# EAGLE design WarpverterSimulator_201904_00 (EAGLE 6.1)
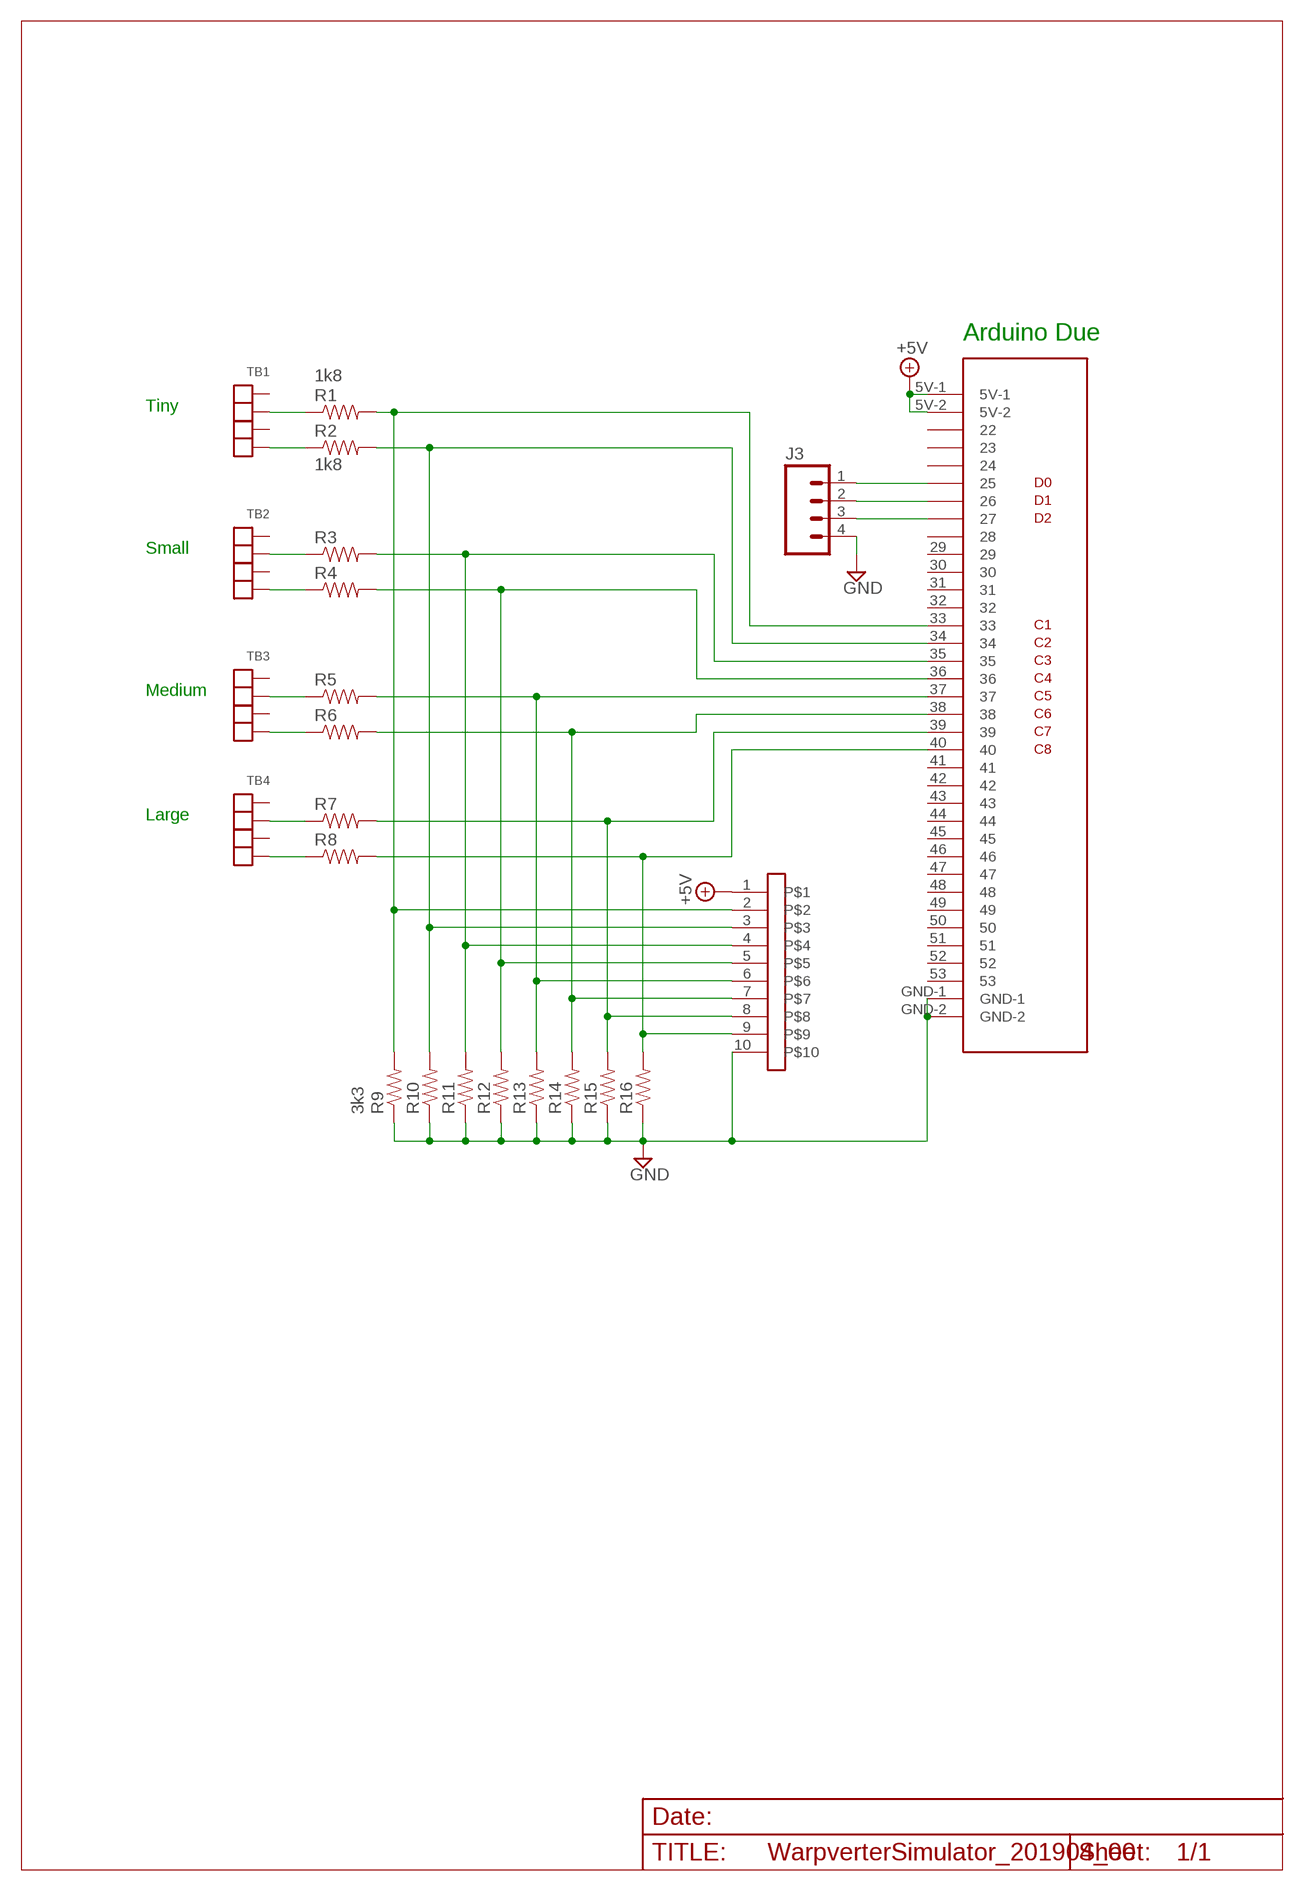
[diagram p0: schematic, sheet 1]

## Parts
J1  DUE-IDC38  [DUE-IDC38]
J2  SIL-STACK-10  [SIL-STACK-10]
J3  SIL4  [SIL4]
R1  1k8  R4  [AXIAL-0.4]
R2  1k8  R4  [AXIAL-0.4]
R3  R4  [AXIAL-0.4]
R4  R4  [AXIAL-0.4]
R5  R4  [AXIAL-0.4]
R6  R4  [AXIAL-0.4]
R7  R4  [AXIAL-0.4]
R8  R4  [AXIAL-0.4]
R9  3k3  R4  [AXIAL-0.4]
R10  R4  [AXIAL-0.4]
R11  R4  [AXIAL-0.4]
R12  R4  [AXIAL-0.4]
R13  R4  [AXIAL-0.4]
R14  R4  [AXIAL-0.4]
R15  R4  [AXIAL-0.4]
R16  R4  [AXIAL-0.4]
TB1  TB4381_SIL  [TB-381-SIL-4P]
TB2  TB4381_SIL  [TB-381-SIL-4P]
TB3  TB4381_SIL  [TB-381-SIL-4P]
TB4  TB4381_SIL  [TB-381-SIL-4P]

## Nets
+5V: J1.5V-1 J1.5V-2 J2.1
GND: J1.GND-1 J1.GND-2 J2.10 J3.4 R9.P$1 R10.P$1 R11.P$1 R12.P$1 R13.P$1 R14.P$1 R15.P$1 R16.P$1
N$1: R1.P$1 TB1.2 TB1.12
N$2: R2.P$1 TB1.4 TB1.14
N$3: R3.P$1 TB2.2 TB2.12
N$4: R4.P$1 TB2.4 TB2.14
N$5: R5.P$1 TB3.2 TB3.12
N$6: R6.P$1 TB3.4 TB3.14
N$7: R7.P$1 TB4.2 TB4.12
N$8: R8.P$1 TB4.4 TB4.14
N$9: J1.33 J2.2 R1.P$2 R9.P$2
N$10: J1.34 J2.3 R2.P$2 R10.P$2
N$11: J1.35 J2.4 R3.P$2 R11.P$2
N$12: J1.36 J2.5 R4.P$2 R12.P$2
N$13: J1.37 J2.6 R5.P$2 R13.P$2
N$14: J1.38 J2.7 R6.P$2 R14.P$2
N$15: J1.39 J2.8 R7.P$2 R15.P$2
N$16: J1.40 J2.9 R8.P$2 R16.P$2
N$18: J1.25 J3.1
N$19: J1.26 J3.2
N$20: J1.27 J3.3
Unconnected: J1.22 J1.23 J1.24 J1.28 J1.29 J1.30 J1.31 J1.32 J1.41 J1.42 J1.43 J1.44 J1.45 J1.46 J1.47 J1.48 J1.49 J1.50 J1.51 J1.52 J1.53 TB1.1 TB1.3 TB1.11 TB1.13 TB2.1 TB2.3 TB2.11 TB2.13 TB3.1 TB3.3 TB3.11 TB3.13 TB4.1 TB4.3 TB4.11 TB4.13

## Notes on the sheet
- Arduino Due
- Tiny
- Small
- Medium
- Large

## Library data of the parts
J1 = Andrew_Arduino:DUE-IDC38
J2 = Andrew_Connectors:SIL-STACK-10
J3 = Andrew_Connectors:SIL4
R1-R16 = Andrew Misc:R4
TB1-TB4 = Andrew_Connectors:TB4

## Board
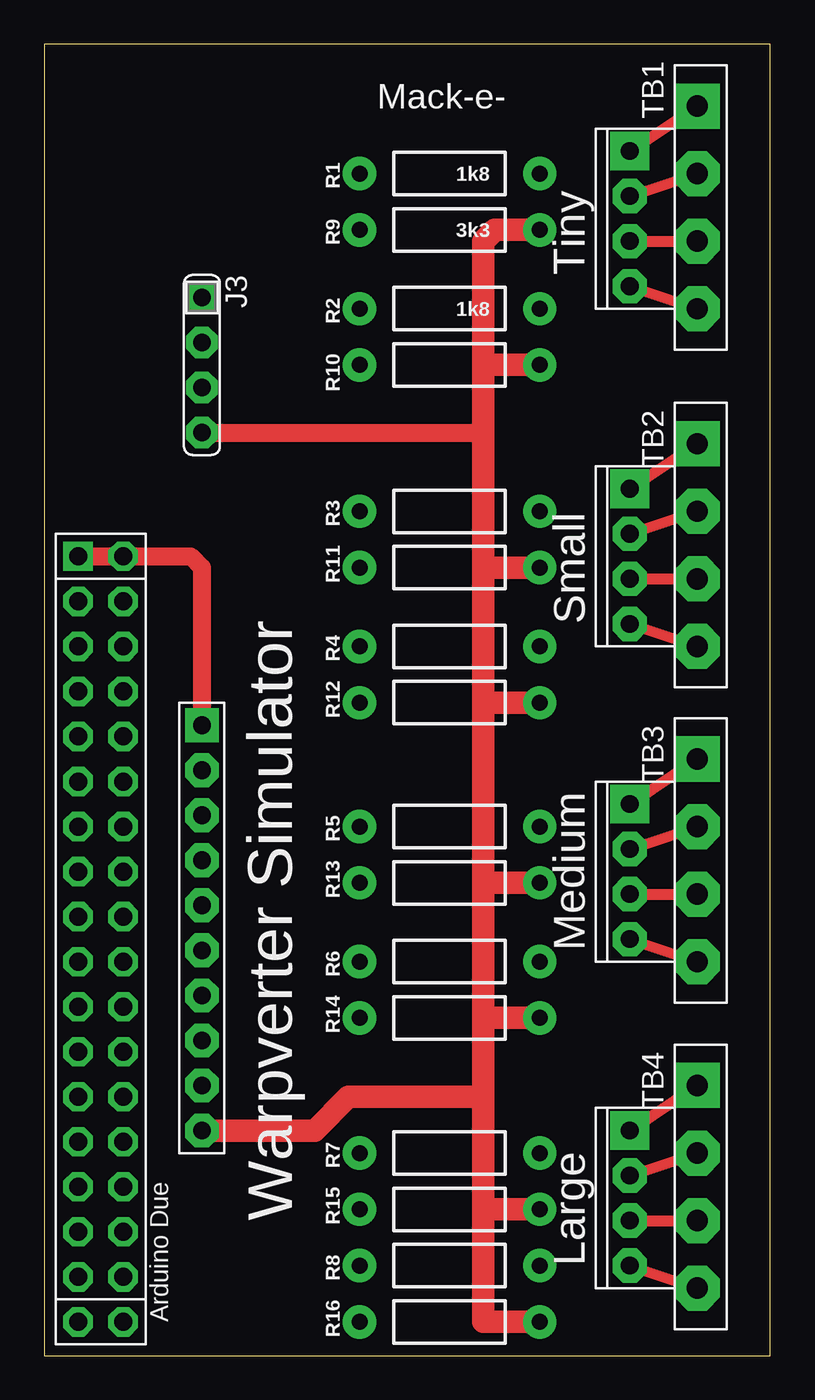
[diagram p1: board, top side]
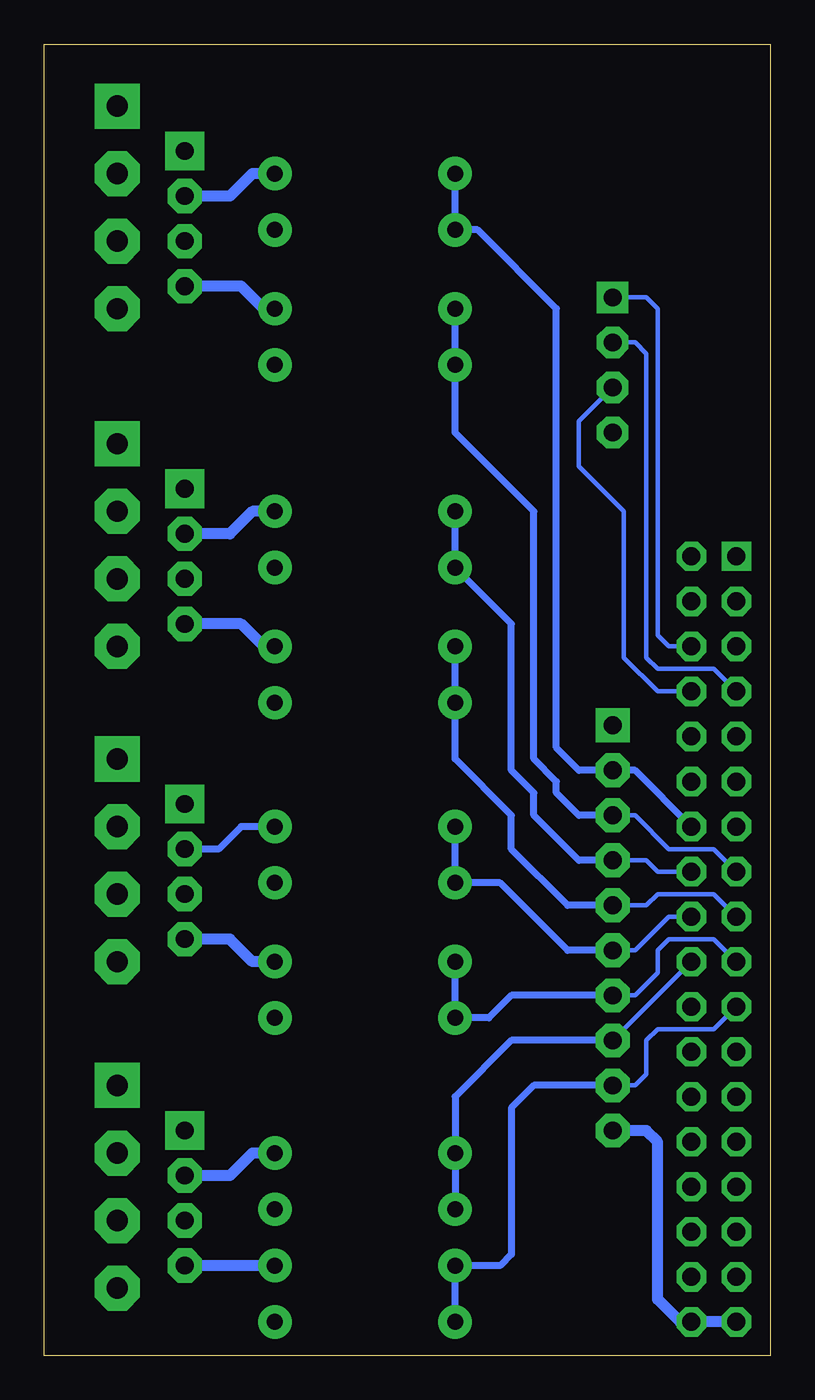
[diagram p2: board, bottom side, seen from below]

Size 40.95 x 73.97 mm. Coordinates in mm from the lower left corner, seen from the top.
Outline: 0,0 40.95,0 40.95,73.97 0,73.97 0,0
Copper layers (1*16): Top 0.035mm / dielectric 1.5mm / Bottom 0.035mm
Design rules: minimum track width 10mil, minimum drill 24mil, track to track 8mil, track to pad 8mil, pad to pad 8mil, via to via 8mil, smd to smd 8mil, copper to edge 40mil, drill to drill 8mil, minimum pad ring 10mil, minimum via ring 8mil, stop-mask expansion 4mil, vias tented up to drill 0mil, thermal gap 10mil

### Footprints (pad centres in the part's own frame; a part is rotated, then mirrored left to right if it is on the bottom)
DUE-IDC38 = drill 1.016 pad 1.651 square: 5V-1 0,2.54 | drill 1.016 pad 1.651 octagon: 5V-2 2.54,2.54; 22 0,0; 23 2.54,0; 24 0,-2.54; 25 2.54,-2.54; 26 0,-5.08; 27 2.54,-5.08; 28 0,-7.62; 29 2.54,-7.62; 30 0,-10.16; 31 2.54,-10.16; 32 0,-12.7; 33 2.54,-12.7; 34 0,-15.24; 35 2.54,-15.24; 36 0,-17.78; 37 2.54,-17.78; 38 0,-20.32; 39 2.54,-20.32; 40 0,-22.86; 41 2.54,-22.86; 42 0,-25.4; 43 2.54,-25.4; 44 0,-27.94; 45 2.54,-27.94; 46 0,-30.48; 47 2.54,-30.48; 48 0,-33.02; 49 2.54,-33.02; 50 0,-35.56; 51 2.54,-35.56; 52 0,-38.1; 53 2.54,-38.1; GND-1 0,-40.64; GND-2 2.54,-40.64
SIL-STACK-10 = drill 1 pad 1.905 square: 1 -11.43,0 | drill 1 pad 1.905 octagon: 2 -8.89,0; 3 -6.35,0; 4 -3.81,0; 5 -1.27,0; 6 1.27,0; 7 3.81,0; 8 6.35,0; 9 8.89,0; 10 11.43,0
SIL4 = drill 1 pad 1.778 square: 1 0,0 | drill 1 pad 1.778 octagon: 2 2.54,0; 3 5.08,0; 4 7.62,0
AXIAL-0.4 = drill 0.9 pad 1.88: P$1 -5.08,0; P$2 5.08,0
TB-381-SIL-4P = drill 1.2 pad 2.54 square: 1 0,0 | drill 1.2 pad 2.54 octagon: 2 3.81,0; 3 7.62,0; 4 11.43,0 | drill 1 pad 2.184 square: 11 2.54,-3.81 | drill 1 pad 1.93 octagon: 12 5.08,-3.81; 13 7.62,-3.81; 14 10.16,-3.81

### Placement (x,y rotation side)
J1  1.91,42.55 0 top
J2  8.89,24.13 270 top
J3  8.89,59.69 270 top
R1  22.86,66.67 180 top
R2  22.86,59.05 180 top
R3  22.86,47.62 180 top
R4  22.86,40.01 180 top
R5  22.86,29.84 180 top
R6  22.86,22.23 180 top
R7  22.86,11.43 180 top
R8  22.86,5.08 180 top
R9  22.86,63.5 180 top
R10  22.86,55.88 180 top
R11  22.86,44.45 180 top
R12  22.86,36.83 180 top
R13  22.86,26.67 180 top
R14  22.86,19.05 180 top
R15  22.86,8.26 180 top
R16  22.86,1.91 180 top
TB1  36.83,70.48 270 top
TB2  36.83,51.44 270 top
TB3  36.83,33.66 270 top
TB4  36.83,15.24 270 top

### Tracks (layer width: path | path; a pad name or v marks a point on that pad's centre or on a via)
+5V
  Top 1.016: J1.5V-1 J1.5V-2 8.26,45.09 8.89,44.45 J2.1
GND
  Top 1.016: J3.4 24.77,52.07
  Top 1.27: R9.P$1 25.4,63.5 24.77,62.87 24.77,55.88 | 24.77,55.88 24.77,52.07 24.77,44.45 | 24.77,44.45 24.77,36.83 | 24.77,36.83 24.77,26.67 | 24.77,26.67 24.77,19.05 | 24.77,19.05 24.77,14.61 | 24.77,14.61 24.77,8.26 | 24.77,8.26 24.77,1.91 R16.P$1 | R15.P$1 24.77,8.26 | R14.P$1 24.77,19.05 | R13.P$1 24.77,26.67 | R12.P$1 24.77,36.83 | R11.P$1 24.77,44.45 | R10.P$1 24.77,55.88 | J2.10 15.24,12.7 17.14,14.61 24.77,14.61
  Bottom 0.61: J1.GND-1 J1.GND-2 5.08,1.91 6.35,3.17 6.35,12.06 6.99,12.7 J2.10
N$1
  Bottom 0.61: R1.P$1 29.21,66.67 30.48,65.41 TB1.12
N$2
  Bottom 0.61: R2.P$1 28.57,59.05 29.84,60.33 TB1.14
N$3
  Bottom 0.61: R3.P$1 29.21,47.62 30.48,46.35 TB2.12
N$4
  Bottom 0.61: R4.P$1 28.57,40.01 29.84,41.27 TB2.14
N$5
  Bottom 0.406: R5.P$1 29.84,29.84 31.11,28.57 TB3.12
N$6
  Bottom 0.61: R6.P$1 29.21,22.23 30.48,23.5 TB3.14
N$7
  Bottom 0.61: R7.P$1 29.21,11.43 30.48,10.16 TB4.12
N$8
  Bottom 0.61: R8.P$1 TB4.14
N$9
  Bottom 0.406: J1.33 7.62,33.02 J2.2 10.79,33.02 12.06,34.29 12.06,59.05 16.51,63.5 R9.P$2 R1.P$2
N$10
  Bottom 0.254: J1.34 3.17,28.57 5.71,28.57 7.62,30.48 J2.3
  Bottom 0.406: J2.3 10.79,30.48 12.06,31.75 12.06,32.38 13.34,33.66 13.34,47.62 17.78,52.07 R10.P$2 R2.P$2
N$11
  Bottom 0.254: J1.35 6.35,27.3 6.99,27.94 J2.4
  Bottom 0.406: J2.4 10.79,27.94 13.34,30.48 13.34,31.75 14.61,33.02 14.61,41.27 R11.P$2 R3.P$2
N$12
  Bottom 0.254: J1.36 3.17,26.04 6.35,26.04 6.99,25.4 J2.5
  Bottom 0.406: J2.5 11.43,25.4 14.61,28.57 14.61,30.48 17.78,33.66 R12.P$2 R4.P$2
N$13
  Bottom 0.254: J1.37 5.71,24.77 7.62,22.86 J2.6
  Bottom 0.406: J2.6 11.43,22.86 15.24,26.67 R13.P$2 R5.P$2
N$14
  Bottom 0.254: J1.38 3.17,23.5 5.71,23.5 6.35,22.86 6.35,21.59 7.62,20.32 J2.7
  Bottom 0.406: J2.7 14.61,20.32 15.88,19.05 R14.P$2 R6.P$2
N$15
  Bottom 0.254: J1.39 J2.8
  Bottom 0.406: J2.8 14.61,17.78 17.78,14.61 R7.P$2 R15.P$2
N$16
  Bottom 0.254: J1.40 3.17,18.41 6.35,18.41 6.99,17.78 6.99,15.88 7.62,15.24 J2.9
  Bottom 0.406: J2.9 13.34,15.24 14.61,13.97 14.61,5.71 15.24,5.08 R8.P$2 R16.P$2
N$18
  Bottom 0.254: J1.25 5.71,40.01 6.35,40.64 6.35,59.05 6.99,59.69 J3.1
N$19
  Bottom 0.254: J1.26 3.17,38.73 6.35,38.73 6.99,39.37 6.99,56.52 7.62,57.15 J3.2
N$20
  Bottom 0.254: J1.27 6.35,37.47 8.26,39.37 8.26,47.62 10.79,50.16 10.79,52.7 J3.3

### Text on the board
tPlace: Mack-e- | Tiny | Small | Medium | Warpverter Simulator | Large | Arduino Due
